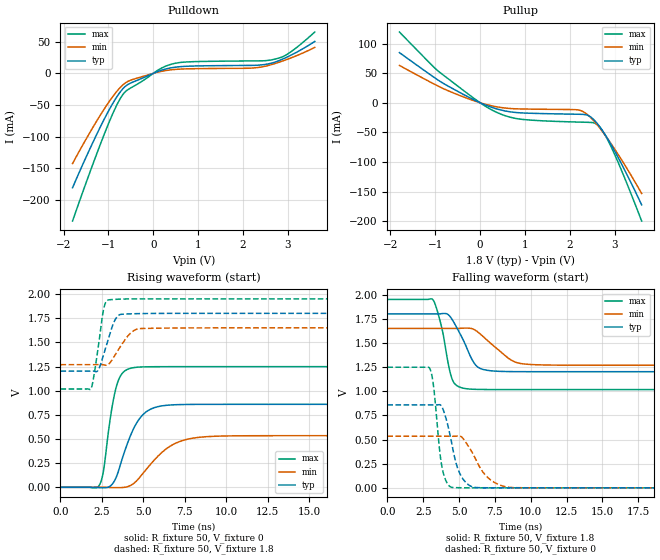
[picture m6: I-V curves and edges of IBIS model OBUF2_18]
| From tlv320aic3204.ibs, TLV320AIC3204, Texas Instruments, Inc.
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[Model]   OBUF2_18
Model_type  Output
Vref =   0
|Rref =   50
Cref =   10p
Vmeas =   0.9
| variable   typ   min   max
C_comp   3.02pF   1.71pF   4.52pF
| C_pullup   3.41pF   1.80pF   4.52pF
| C_pulldown   2.63pF   1.71pF   3.35pF
[Temperature Range]   40   100   -40
| Ambient temperature   25   85   -40
[Voltage range]   1.8   1.65   1.95
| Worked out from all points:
|   slope of the pulldown table from 0 to 0.27 V, typ, clamps not added: 40.3 ohm
|   slope of the pullup table from 0 to 0.27 V, typ, clamps not added: 33.7 ohm
|   rising waveform, R_fixture 50, V_fixture 0: 20-80 % time 1.17ns typ, 1.84ns min, 645ps max; typ from 0 V to 0.859 V
|   falling waveform, R_fixture 50, V_fixture 1.8: 20-80 % time 1.17ns typ, 1.79ns min, 752ps max; typ from 1.8 V to 1.2 V
|   rising waveform, R_fixture 50, V_fixture 1.8: 20-80 % time 647ps typ, 896ps min, 459ps max; typ from 1.2 V to 1.8 V
|   falling waveform, R_fixture 50, V_fixture 0: 20-80 % time 837ps typ, 1.34ns min, 506ps max; typ from 0.859 V to 0 V
[Pulldown]
| OBUF2_18
|   Voltage   I(typ)   I(min)   I(max)
-1.8V     -180.5mA   -142.4mA   -233mA
-1.35V    -109.5mA   -85.67mA   -143.9mA
-985mV    -57.7mA    -44.71mA   -77.08mA
-755mV    -31.1mA    -23.68mA   -42.09mA
-590mV    -18.72mA   -13.65mA   -26.96mA
145mV     4.06mA     2.627mA    6.836mA
480mV     9.604mA    6.154mA    15.76mA
2.21V     12.56mA    8.381mA    19.62mA
2.545V    14.71mA    12.08mA    20.28mA
2.81V     20.29mA    17.68mA    24.33mA
3.1V      29.76mA    25.16mA    35.64mA
3.6V      50.32mA    40.92mA    65.19mA
[Pullup]
| OBUF2_18
|   Voltage   I(typ)   I(min)   I(max)
-1.8V     84.79mA    63.13mA    119.6mA
-935mV    38.21mA    28.13mA    53.53mA
-150mV    5.403mA    3.727mA    8.185mA
350mV     -9.912mA   -6.53mA    -15.51mA
910mV     -17.05mA   -10.44mA   -27.79mA
2.19V     -19.37mA   -12.2mA    -32.61mA
2.42V     -22.01mA   -21.84mA   -33.06mA
2.61V     -35.02mA   -37.29mA   -36.9mA
2.76V     -50.92mA   -52.02mA   -51.36mA
2.96V     -76.31mA   -73.85mA   -80.91mA
3.23V     -115mA     -105.8mA   -128.7mA
3.6V      -172.6mA   -153.3mA   -199.8mA
[Ramp]
| OBUF2_18
| variable   typ   min   max
dV/dt_r   0.52/1.17E-09   0.32/1.85E-09   0.75/6.50E-10
dV/dt_f   0.36/1.18E-09   0.23/1.81E-09   0.56/7.61E-10
R_load = 50
[Rising Waveform]
| OBUF2_18
R_fixture =   50
C_fixture =   0
L_fixture =   0
V_fixture =   0
V_fixture_min = 0
V_fixture_max = 0
|   Time   V(typ)   V(min)   V(max)
0s        1.776nV    16.92nV    626.2pV
2.335ns   -3.593mV   -25.68uV   19.42mV
2.58ns    -4.953mV   311uV      156.2mV
3.055ns   20.35mV    -3.006mV   770.4mV
3.42ns    129.5mV    -3.852mV   1.071V
4.565ns   657.4mV    62.35mV    1.242V
5.38ns    803.9mV    227.9mV    1.247V
6.69ns    852.4mV    433.4mV    1.248V
9.225ns   858.6mV    527.7mV    1.248V
70ns      858.8mV    534.2mV    1.248V
[Falling Waveform]
| OBUF2_18
R_fixture =   50
C_fixture =   0
L_fixture =   0
V_fixture =   1.8
V_fixture_min = 1.65
V_fixture_max = 1.95
|   Time   V(typ)   V(min)   V(max)
0s        1.8V       1.65V      1.95V
3.175ns   1.8V       1.65V      1.948V
3.76ns    1.802V     1.65V      1.68V
4.53ns    1.74V      1.65V      1.122V
5.665ns   1.404V     1.653V     1.024V
6.135ns   1.276V     1.631V     1.02V
6.64ns    1.227V     1.572V     1.018V
8.71ns    1.203V     1.316V     1.017V
10.33ns   1.202V     1.274V     1.017V
70ns      1.202V     1.269V     1.017V
[Rising Waveform]
| OBUF2_18
R_fixture =   50
C_fixture =   0
L_fixture =   0
V_fixture =   1.8
V_fixture_min = 1.65
V_fixture_max = 1.95
|   Time   V(typ)   V(min)   V(max)
0s        1.202V     1.269V     1.017V
1.835ns   1.202V     1.269V     1.018V
2.25ns    1.207V     1.269V     1.417V
2.605ns   1.375V     1.267V     1.845V
2.775ns   1.471V     1.263V     1.927V
3.015ns   1.606V     1.295V     1.942V
3.53ns    1.782V     1.434V     1.947V
4.29ns    1.795V     1.605V     1.949V
4.985ns   1.798V     1.644V     1.95V
70ns      1.8V       1.65V      1.95V
[Falling Waveform]
| OBUF2_18
R_fixture =   50
C_fixture =   0
L_fixture =   0
V_fixture =   0
V_fixture_min = 0
V_fixture_max = 0
|   Time   V(typ)   V(min)   V(max)
0s        858.8mV    534.2mV    1.248V
2.955ns   858.8mV    534.2mV    1.237V
3.22ns    858.7mV    534.2mV    1.057V
3.82ns    835.2mV    534.2mV    209.2mV
4.54ns    424.5mV    534mV      3.619mV
5.005ns   165.5mV    536.9mV    1.33mV
5.685ns   28.39mV    423mV      322.1uV
6.99ns    919.6uV    109.1mV    29.12uV
8.695ns   84.03uV    3.033mV    2.366uV
70ns      1.694nV    15.86nV    460.2pV
